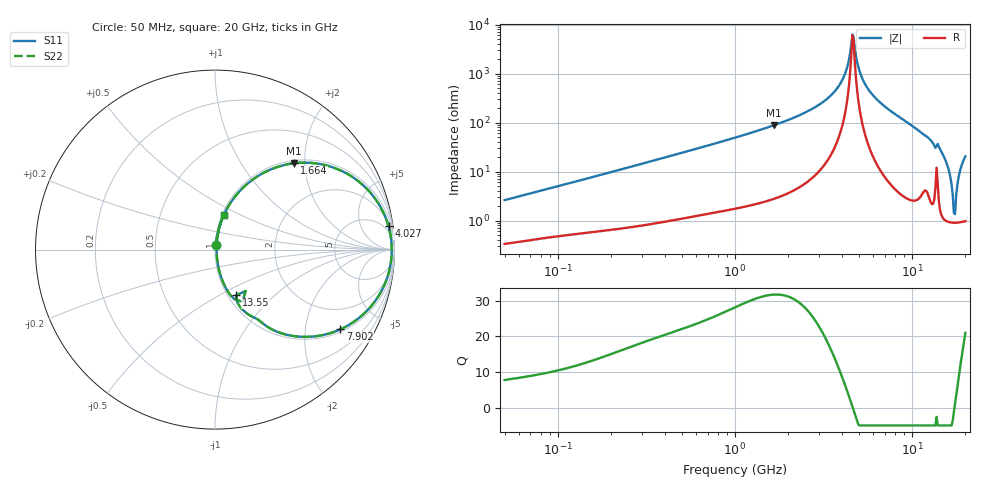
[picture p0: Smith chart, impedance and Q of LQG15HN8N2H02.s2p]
!Murata Part Number: LQG15HN8N2H02
!These Parameters are Measured in Series Mode Connection
!  o--[Z]--o
!Port1  Port2
!  o-------o
!Freq. Start=50[MHz] Stop=20[GHz], 401[Steps]
# Hz S RI R 50
!Freq.(Hz) S11(Real) S11(Imag) S21(Real) S21(Imag) S12(Real) S12(Imag) S22(Real) S22(Imag)
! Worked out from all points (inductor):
!   401 points, 50 MHz to 20 GHz, reference 50 ohm
!   read as one part in series: L = 8.14 nH near 51.52 MHz
!   highest Q = 31.8 at 1.664 GHz (marker M1), where L = 8.46 nH
!   self-resonance near 4.608 GHz
!   S11 on the Smith chart (normalised r, x): 50 MHz: 1.01, +0.05; 1.664 GHz: 1.06, +1.77; 4.027 GHz: 3, +14; 7.902 GHz: 1.09, -3.08; 13.55 GHz: 1.09, -0.60; 20 GHz: 1.02, +0.41
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5e7  0.00399 0.0257  0.996 -0.0257  0.996 -0.0257  0.00399 0.0257
1.364002e8  0.00989 0.0663  0.9901 -0.0663  0.9901 -0.0663  0.00989 0.0663
3.721004e8  0.0394 0.1709  0.9606 -0.1709  0.9606 -0.1709  0.0394 0.1709
1e9  0.2029 0.3848  0.7971 -0.3848  0.7971 -0.3848  0.2029 0.3848
1.664083e9  0.441 0.481  0.559 -0.481  0.559 -0.481  0.441 0.481
2.728004e9  0.7745 0.3989  0.2255 -0.3989  0.2255 -0.3989  0.7745 0.3989
3.466789e9  0.9127 0.2535  0.0873 -0.2535  0.0873 -0.2535  0.9127 0.2535
4.026975e9  0.9669 0.13  0.0331 -0.13  0.0331 -0.13  0.9669 0.13
4.275624e9  0.9789 0.0754  0.0211 -0.0754  0.0211 -0.0754  0.9789 0.0754
4.539627e9  0.9845 0.0187  0.0155 -0.0187  0.0155 -0.0187  0.9845 0.0187
4.677679e9  0.9849 -0.0101  0.0151 0.0101  0.0151 0.0101  0.9849 -0.0101
5.041459e9  0.978 -0.083  0.022 0.083  0.022 0.083  0.978 -0.083
5.433528e9  0.9598 -0.1556  0.0402 0.1556  0.0402 0.1556  0.9598 -0.1556
7.442007e9  0.7578 -0.4126  0.2422 0.4126  0.2422 0.4126  0.7578 -0.4126
7.901521e9  0.6985 -0.4443  0.3015 0.4443  0.3015 0.4443  0.6985 -0.4443
1.034674e10  0.3859 -0.4708  0.6141 0.4708  0.6141 0.4708  0.3859 -0.4708
1.354865e10  0.1181 -0.254  0.8819 0.254  0.8819 0.254  0.1181 -0.254
1.573793e10  0.0284 -0.1353  0.9716 0.1353  0.9716 0.1353  0.0284 -0.1353
1.721783e10  0.00907 -0.011  0.9909 0.011  0.9909 0.011  0.00907 -0.011
1.774144e10  0.00992 0.0308  0.9901 -0.0308  0.9901 -0.0308  0.00992 0.0308
1.88369e10  0.0223 0.1134  0.9777 -0.1134  0.9777 -0.1134  0.0223 0.1134
2e10  0.0488 0.1929  0.9512 -0.1929  0.9512 -0.1929  0.0488 0.1929
